(* Logix 5000 AddOnInstructionDefinition export Banner_iVu_VE_Functions; software revision 33.00 *)

TYPE Banner_iVu_VE_Control :   // Tags that control some basic functions of iVu and VE units.
STRUCT
   Reserved_PC : BOOL;   // Reserved for AOI internal use, to write to the VE input bit, for changing the running Inspection
   Reserved_TL : BOOL;   // Reserved for AOI internal use, to write to the VE input bit, For Match Teach, or Barcode Data Compare Teach
   Reserved_TR : BOOL;   // Reserved for AOI internal use, to write to the VE input bit, For triggering an image acquisition
   iVu_Command : BOOL;   // For iVu Command Channel over EIP only
   VE_Barcode_Data_Compare_Input_String : BOOL;   // For VE Barcode Data Compare only, saves a new compare string
   VE_FTP_Input_String : BOOL;   // For VE FTP file naming only, sends a new filename string
END_STRUCT
END_TYPE

TYPE Banner_iVu_VE_Data :   // Banner iVu and VE function data
STRUCT
   DTI : INT[17];   // Data Input Transfer Array
   DTO : INT[34];   // Data Output Transfer Array
   In : Banner_iVu_VE_Inputs;   // Input Data
   Out : Banner_iVu_VE_Outputs;   // Output Data
   Product_Change : BOOL;   // Tag that controls when a product change should be activated.
   Request_Product_Num : DINT;   // Tag in which the requested product change number is entered.
   Product_Change_Error : BOOL;   // Tag that states when a product change error has occurred.
   Teach : BOOL;   // Tag that controls when a teach should be activated.
   Teach_Request_Error : BOOL;   // Tag that states when a teach request error has occurred.
   Trigger : BOOL;   // Tag that controls when a trigger should be activated.
   Continuous_Trigger : BOOL;   // Tag that controls if triggering will be continuous or not.
   Trigger_Error : BOOL;   // Tag that states when a trigger error has occurred.
END_STRUCT
END_TYPE

TYPE Banner_iVu_VE_Input_Bits_Ack :
STRUCT
   Product_Change_Ack : BOOL;
   Teach_Latch_Ack : BOOL;
   Trigger_Ack : BOOL;
   iVu_Command_Ack : BOOL;
   VE_Barcode_Data_Compare_Input_String_Ack : BOOL;
   VE_FTP_Input_String_Ack : BOOL;
END_STRUCT
END_TYPE

TYPE Banner_iVu_VE_Inputs :
STRUCT
   Input_Bits_Ack : Banner_iVu_VE_Input_Bits_Ack;
   Output_Bits_Status : Banner_iVu_VE_Output_Status;
   Error_Code : DINT;
   Inspection_Num : DINT;
   Iteration_Count : DINT;
   Pass_Count : DINT;
   Fail_Count : DINT;
   Missed_Triggers : DINT;
   Current_Inspection_Time : REAL;
   Sensor_Pass_Fail : INT;
END_STRUCT
END_TYPE

TYPE Banner_iVu_VE_Output_Status :
STRUCT
   Ready : BOOL;
   Pass_Fail : BOOL;
   Read_No_Read_iVu : BOOL;   // (iVu BCR Only)
   Ready_to_Latch : BOOL;
   Output_1 : BOOL;
   Output_2 : BOOL;
   Output_3 : BOOL;
   Output_4_VE : BOOL;   // (VE Only)
   Output_5_VE : BOOL;   // (VE Only)
   Missed_Trigger : BOOL;
   Teach_Error : BOOL;
   System_Error : BOOL;
   Execution_Error : BOOL;
END_STRUCT
END_TYPE

TYPE Banner_iVu_VE_Outputs :
STRUCT
   Control_Registers : Banner_iVu_VE_Control;
   Reserved_PCN : DINT;   // Reserved for AOI Internal Use, to write the VE input value, for the requested product change inspection number
   VE_Input_String_Tool_Index : SINT;   // Specifies which Barcode tool in the VE Inspection should receive the string data (Optional)
   VE_Input_String : STRING_26;   // String for using as the barcode tool data compare Test string, or an FTP image file name
END_STRUCT
END_TYPE

TYPE STRING_26 :   // string type
STRUCT
   LEN : DINT;
   DATA : SINT[26];
END_STRUCT
END_TYPE

ADD_ON_INSTRUCTION Banner_iVu_VE_Convert_Data   (* revision 1.0 *)
VAR_IN_OUT
   Data : Banner_iVu_VE_Data; {required}
END_VAR

ROUTINE Logic   (* ladder *)
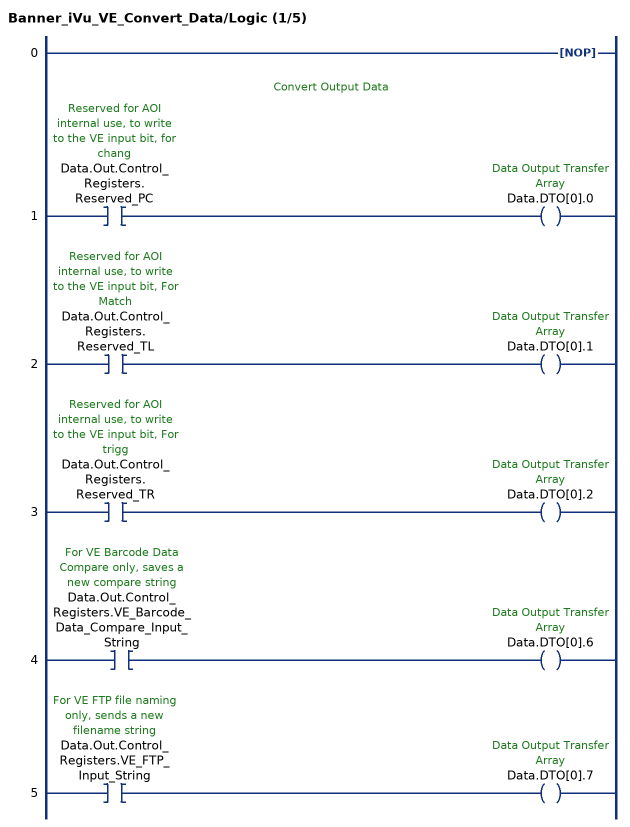
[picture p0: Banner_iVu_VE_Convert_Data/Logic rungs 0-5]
   0: NOP();
   // Convert Output Data
   1: XIC(Data.Out.Control_Registers.Reserved_PC)OTE(Data.DTO[0].0);
   2: XIC(Data.Out.Control_Registers.Reserved_TL)OTE(Data.DTO[0].1);
   3: XIC(Data.Out.Control_Registers.Reserved_TR)OTE(Data.DTO[0].2);
   4: XIC(Data.Out.Control_Registers.VE_Barcode_Data_Compare_Input_String)OTE(Data.DTO[0].6);
   5: XIC(Data.Out.Control_Registers.VE_FTP_Input_String)OTE(Data.DTO[0].7);
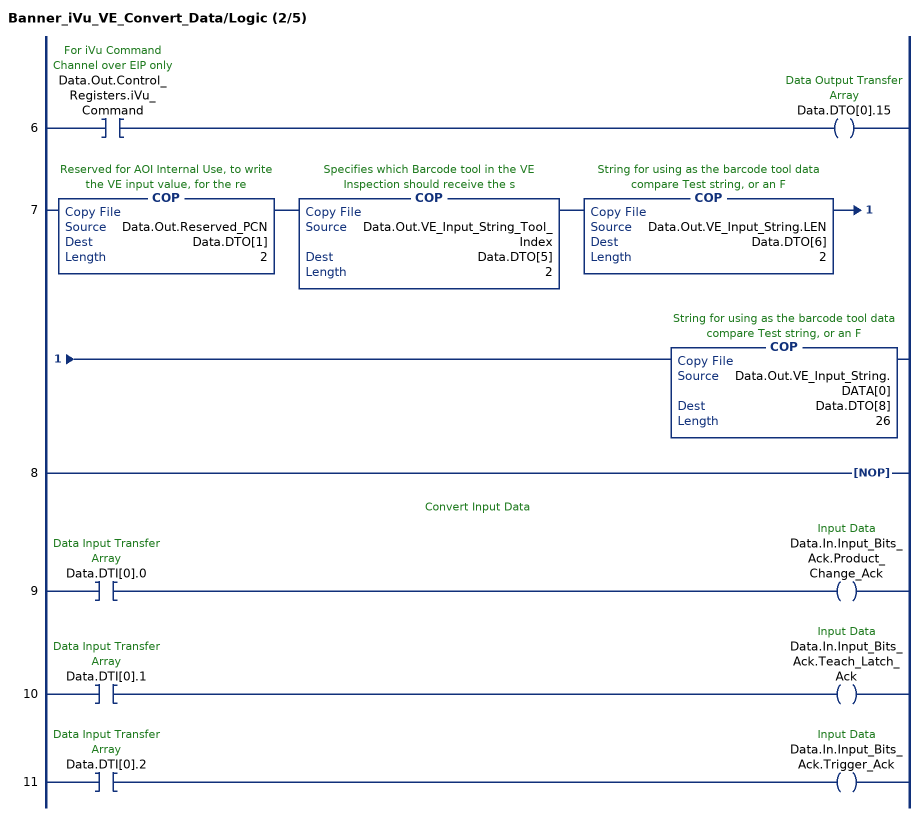
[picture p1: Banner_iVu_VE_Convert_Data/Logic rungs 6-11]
   6: XIC(Data.Out.Control_Registers.iVu_Command)OTE(Data.DTO[0].15);
   7: COP(Data.Out.Reserved_PCN,Data.DTO[1],2)COP(Data.Out.VE_Input_String_Tool_Index,Data.DTO[5],2)COP(Data.Out.VE_Input_String.LEN,Data.DTO[6],2)COP(Data.Out.VE_Input_String.DATA[0],Data.DTO[8],26);
   8: NOP();
   // Convert Input Data
   9: XIC(Data.DTI[0].0)OTE(Data.In.Input_Bits_Ack.Product_Change_Ack);
   10: XIC(Data.DTI[0].1)OTE(Data.In.Input_Bits_Ack.Teach_Latch_Ack);
   11: XIC(Data.DTI[0].2)OTE(Data.In.Input_Bits_Ack.Trigger_Ack);
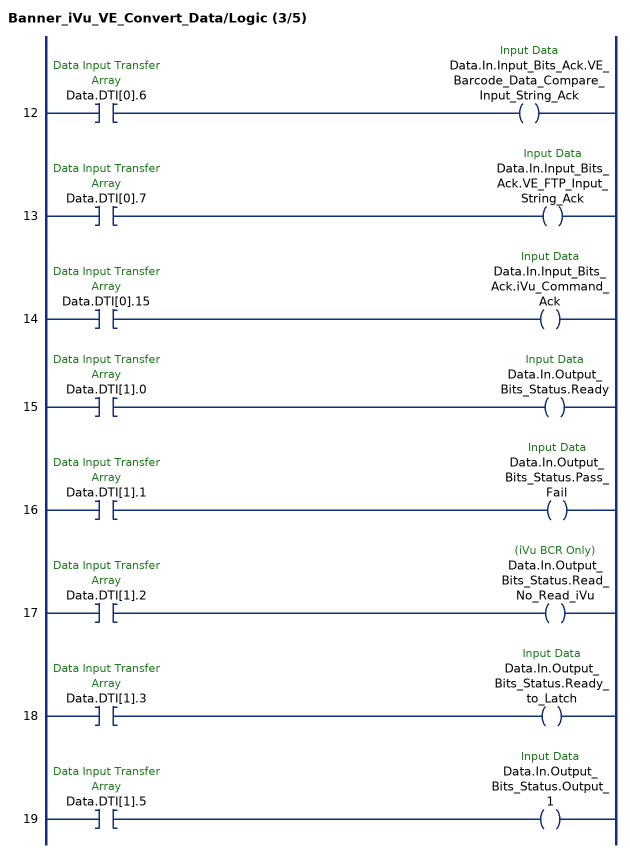
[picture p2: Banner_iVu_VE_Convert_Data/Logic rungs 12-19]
   12: XIC(Data.DTI[0].6)OTE(Data.In.Input_Bits_Ack.VE_Barcode_Data_Compare_Input_String_Ack);
   13: XIC(Data.DTI[0].7)OTE(Data.In.Input_Bits_Ack.VE_FTP_Input_String_Ack);
   14: XIC(Data.DTI[0].15)OTE(Data.In.Input_Bits_Ack.iVu_Command_Ack);
   15: XIC(Data.DTI[1].0)OTE(Data.In.Output_Bits_Status.Ready);
   16: XIC(Data.DTI[1].1)OTE(Data.In.Output_Bits_Status.Pass_Fail);
   17: XIC(Data.DTI[1].2)OTE(Data.In.Output_Bits_Status.Read_No_Read_iVu);
   18: XIC(Data.DTI[1].3)OTE(Data.In.Output_Bits_Status.Ready_to_Latch);
   19: XIC(Data.DTI[1].5)OTE(Data.In.Output_Bits_Status.Output_1);
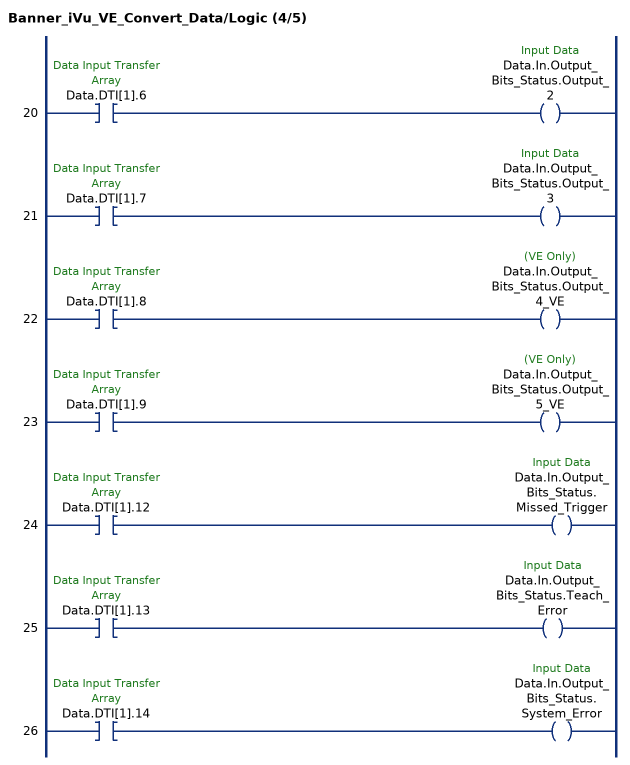
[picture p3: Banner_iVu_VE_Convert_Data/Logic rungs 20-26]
   20: XIC(Data.DTI[1].6)OTE(Data.In.Output_Bits_Status.Output_2);
   21: XIC(Data.DTI[1].7)OTE(Data.In.Output_Bits_Status.Output_3);
   22: XIC(Data.DTI[1].8)OTE(Data.In.Output_Bits_Status.Output_4_VE);
   23: XIC(Data.DTI[1].9)OTE(Data.In.Output_Bits_Status.Output_5_VE);
   24: XIC(Data.DTI[1].12)OTE(Data.In.Output_Bits_Status.Missed_Trigger);
   25: XIC(Data.DTI[1].13)OTE(Data.In.Output_Bits_Status.Teach_Error);
   26: XIC(Data.DTI[1].14)OTE(Data.In.Output_Bits_Status.System_Error);
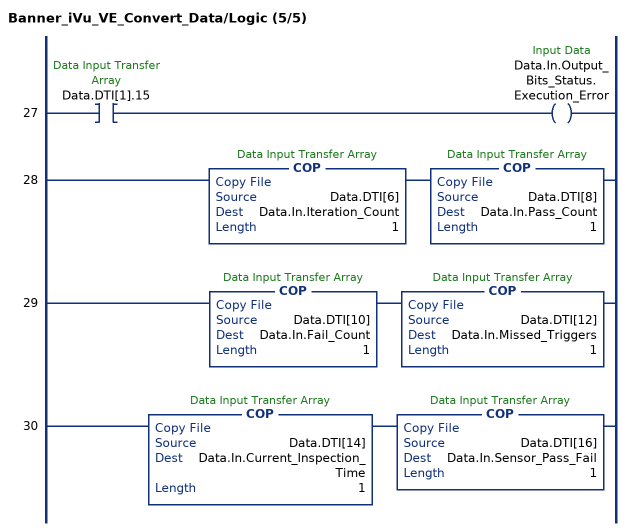
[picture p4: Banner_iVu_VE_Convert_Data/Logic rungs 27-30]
   27: XIC(Data.DTI[1].15)OTE(Data.In.Output_Bits_Status.Execution_Error);
   28: COP(Data.DTI[6],Data.In.Iteration_Count,1)COP(Data.DTI[8],Data.In.Pass_Count,1);
   29: COP(Data.DTI[10],Data.In.Fail_Count,1)COP(Data.DTI[12],Data.In.Missed_Triggers,1);
   30: COP(Data.DTI[14],Data.In.Current_Inspection_Time,1)COP(Data.DTI[16],Data.In.Sensor_Pass_Fail,1);
END_ROUTINE
END_ADD_ON_INSTRUCTION

ADD_ON_INSTRUCTION Banner_Vision_Product_Change   (* revision 1.0, vendor Banner Engineering *)
// Instruction to do a product change for a iVu or VE vision sensor.
VAR_INPUT
   Ready_Bit : BOOL; {required}   // Bit that determines status of the Vision Sensor.
   Product_Change_ACK_Bit : BOOL; {required}   // Bit that states the Acknowledgement Bit Status.
   Requested_Product_Number : INT; {required}   // Product Number that the PLC is requesting.
   System_Error_Bit : BOOL; {required}   // Status of the System Error Bit.
   Execution_Error_Bit : BOOL; {required}   // Status of the Execution Error Bit.
END_VAR
VAR_IN_OUT
   Error_Output : BOOL; {required}   // If the Product Change fails activate an Error Bit so the PLC can solve the error.
   Product_Change_Bit : BOOL; {required}   // Bit that controls the Product Change proces.
   Product_Change_Control_Bit : BOOL; {required}   // Bit that controls the Product Change routine.
   Product_Change_Number : DINT; {required}   // Inspection number that the Vision sensor should change to.
END_VAR
VAR
   Lock_2 : BOOL; {access None}
   Ladder_Control_Bit : BOOL; {access None}
   Timer : TIMER := (PRE := 50); {access None}
END_VAR

ROUTINE Logic   (* ladder *)
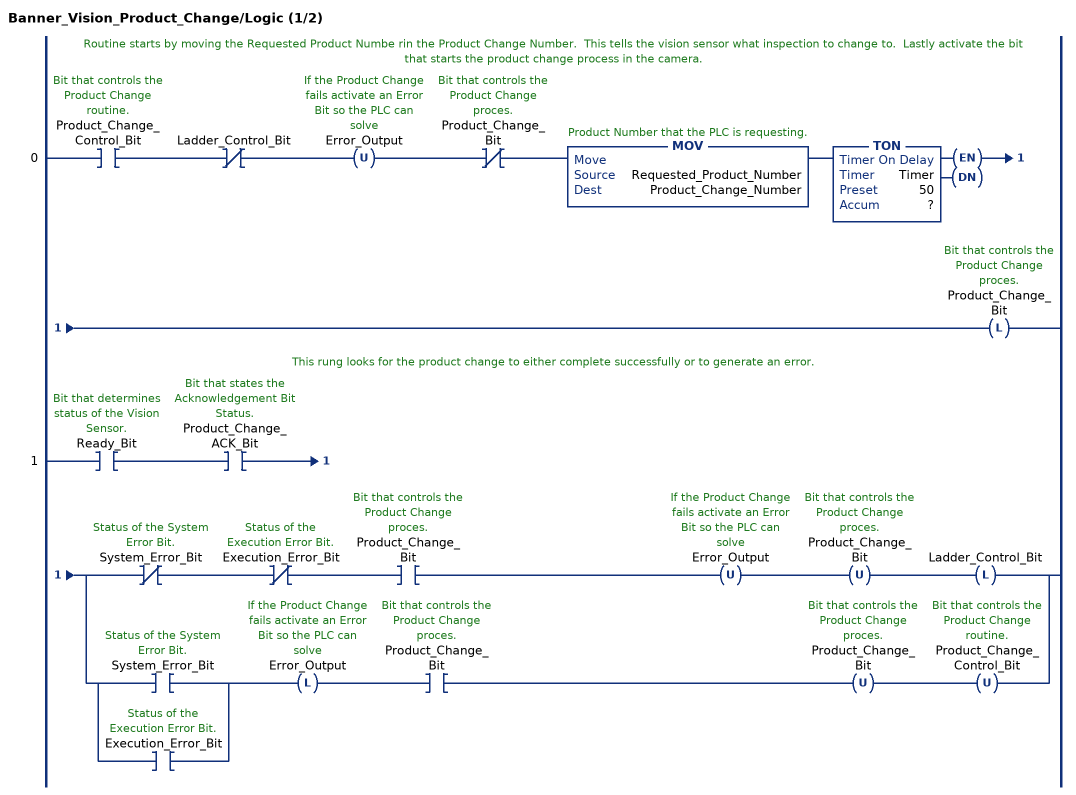
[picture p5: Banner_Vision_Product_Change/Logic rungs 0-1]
   // Routine starts by moving the Requested Product Numbe rin the Product Change Number.  This tells the vision sensor what inspection to change to.  Lastly activate the bit that starts the product change process in the camera.
   0: XIC(Product_Change_Control_Bit)XIO(Ladder_Control_Bit)OTU(Error_Output)XIO(Product_Change_Bit)MOV(Requested_Product_Number,Product_Change_Number)TON(Timer,?,?)OTL(Product_Change_Bit);
   // This rung looks for the product change to either complete successfully or to generate an error.
   1: XIC(Ready_Bit)XIC(Product_Change_ACK_Bit)[XIO(System_Error_Bit) XIO(Execution_Error_Bit) XIC(Product_Change_Bit) OTU(Error_Output) OTU(Product_Change_Bit) OTL(Ladder_Control_Bit) ,[XIC(System_Error_Bit) ,XIC(Execution_Error_Bit) ] OTL(Error_Output) XIC(Product_Change_Bit) OTU(Product_Change_Bit) OTU(Product_Change_Control_Bit) ];
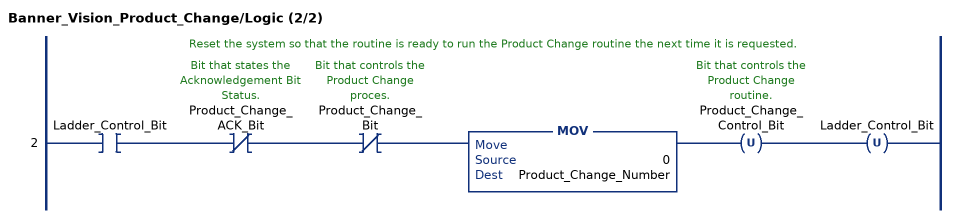
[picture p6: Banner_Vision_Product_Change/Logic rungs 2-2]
   // Reset the system so that the routine is ready to run the Product Change routine the next time it is requested.
   2: XIC(Ladder_Control_Bit)XIO(Product_Change_ACK_Bit)XIO(Product_Change_Bit)MOV(0,Product_Change_Number)OTU(Product_Change_Control_Bit)OTU(Ladder_Control_Bit);
END_ROUTINE
END_ADD_ON_INSTRUCTION

ADD_ON_INSTRUCTION Banner_Vision_Teach   (* revision 1.0, vendor Banner Engineering *)
// Instruction to request a Teach for a iVu or VE vision sensor.
VAR_INPUT
   Teach_Ack_Bit : BOOL; {required}   // Status of the Teach Acknowledgement bit.
   Ready_Bit : BOOL; {required}   // Status of the Camera Ready bit.
   Execution_Error : BOOL; {required}   // Status of the Execution Error from the Vision Sensor.
   System_Error : BOOL; {required}   // Status of the System Error from the Vision Sensor.
   Teach_Error : BOOL; {required}   // Status of the Teach Error from the Vision Sensor.
END_VAR
VAR_IN_OUT
   Teach_Error_Output : BOOL; {required}   // When an error in the Teach routine is detected activated this bit so the PLC can begin a recovery routine.
   Teach_Control_Bit : BOOL; {required}   // Bit that controls the activation of the Teach AOI.
   Teach_Bit : BOOL; {required}   // Bit that controls the activation of the Teach routine in the vision sensor.
END_VAR
VAR
   Ladder_Control_2 : BOOL; {access None}
   Ladder_Control_1 : BOOL; {access None}
END_VAR

ROUTINE Logic   (* ladder *)
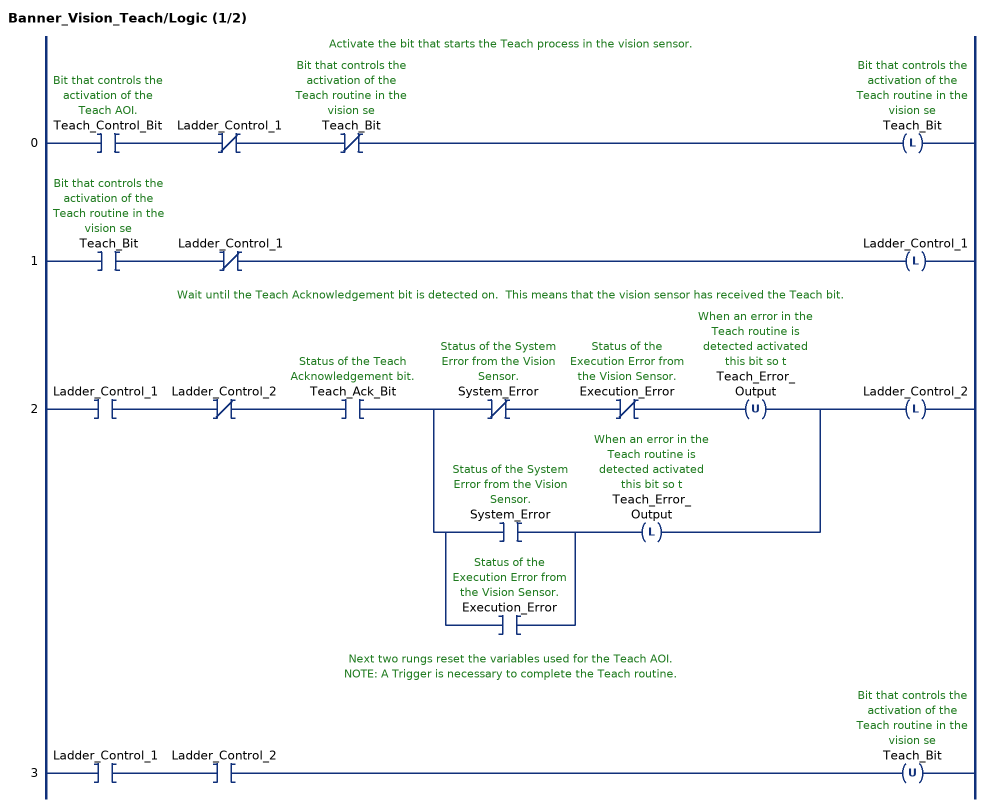
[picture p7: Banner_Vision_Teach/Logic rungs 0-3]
   // Activate the bit that starts the Teach process in the vision sensor.
   0: XIC(Teach_Control_Bit)XIO(Ladder_Control_1)XIO(Teach_Bit)OTL(Teach_Bit);
   1: XIC(Teach_Bit)XIO(Ladder_Control_1)OTL(Ladder_Control_1);
   // Wait until the Teach Acknowledgement bit is detected on.  This means that the vision sensor has received the Teach bit.
   2: XIC(Ladder_Control_1)XIO(Ladder_Control_2)XIC(Teach_Ack_Bit)[XIO(System_Error) XIO(Execution_Error) OTU(Teach_Error_Output) ,[XIC(System_Error) ,XIC(Execution_Error) ] OTL(Teach_Error_Output) ]OTL(Ladder_Control_2);
   // Next two rungs reset the variables used for the Teach AOI.
   // NOTE: A Trigger is necessary to complete the Teach routine.
   3: XIC(Ladder_Control_1)XIC(Ladder_Control_2)OTU(Teach_Bit);
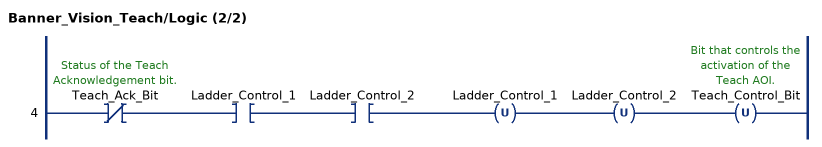
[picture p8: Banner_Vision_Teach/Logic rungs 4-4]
   4: XIO(Teach_Ack_Bit)XIC(Ladder_Control_1)XIC(Ladder_Control_2)OTU(Ladder_Control_1)OTU(Ladder_Control_2)OTU(Teach_Control_Bit);
END_ROUTINE
END_ADD_ON_INSTRUCTION

ADD_ON_INSTRUCTION Banner_Vision_Trigger   (* revision 1.0, vendor Banner Engineering *)
// Instruction to do a Trigger for a iVu or VE vision sensor.
VAR_INPUT
   Ready_Bit : BOOL; {required}   // Status of the Ready Bit from the Vision Sensor.
   Trigger_Ack_Bit : BOOL; {required}   // Status of the Trigger Acknowledgement Bit.
   System_Error : BOOL; {required}   // Status of the System Error from the Vision Sensor.
   Execution_Error : BOOL; {required}   // Status of the Execution Error from the Vision Sensor.
END_VAR
VAR_IN_OUT
   Trigger_Error : BOOL; {required}   // The Trigger Error bit is activated when the AOI detects an error from the Vision Sensor.
   Trigger_Bit : BOOL; {required}   // Trigger Bit controls the activation of a Trigger in the Vision Sensor.
   Trigger_Control : BOOL; {required}   // Bit that controls the activation of the Vision Trigger AOI.
END_VAR
VAR
   Ladder_Control : BOOL; {access None}
END_VAR

ROUTINE Logic   (* ladder *)
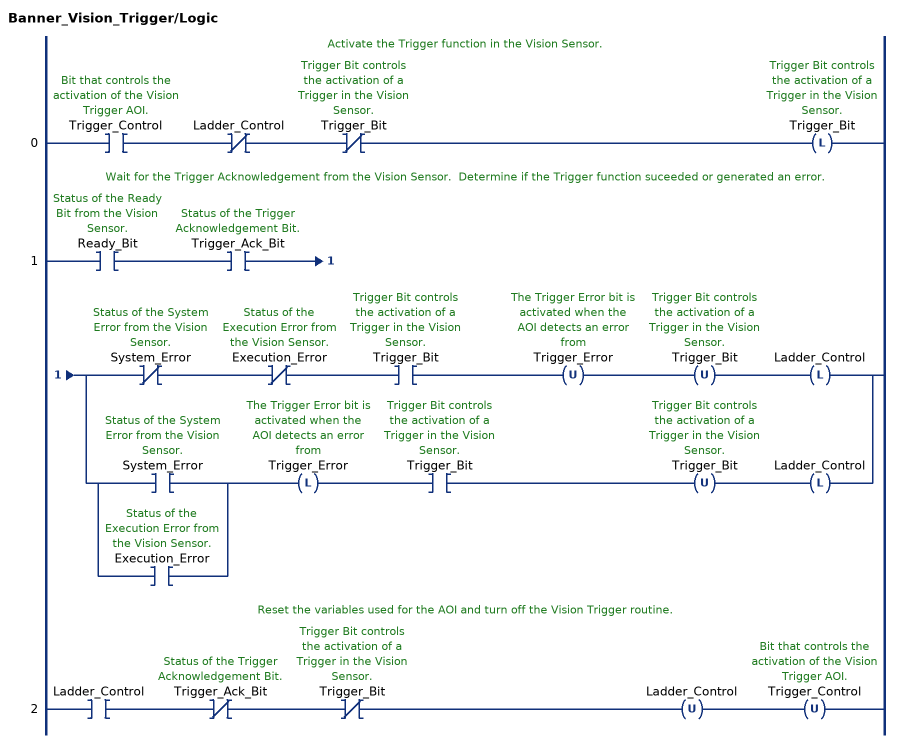
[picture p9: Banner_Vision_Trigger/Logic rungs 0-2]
   // Activate the Trigger function in the Vision Sensor.
   0: XIC(Trigger_Control)XIO(Ladder_Control)XIO(Trigger_Bit)OTL(Trigger_Bit);
   // Wait for the Trigger Acknowledgement from the Vision Sensor.  Determine if the Trigger function suceeded or generated an error.
   1: XIC(Ready_Bit)XIC(Trigger_Ack_Bit)[XIO(System_Error) XIO(Execution_Error) XIC(Trigger_Bit) OTU(Trigger_Error) OTU(Trigger_Bit) OTL(Ladder_Control) ,[XIC(System_Error) ,XIC(Execution_Error) ] OTL(Trigger_Error) XIC(Trigger_Bit) OTU(Trigger_Bit) OTL(Ladder_Control) ];
   // Reset the variables used for the AOI and turn off the Vision Trigger routine.
   2: XIC(Ladder_Control)XIO(Trigger_Ack_Bit)XIO(Trigger_Bit)OTU(Ladder_Control)OTU(Trigger_Control);
END_ROUTINE
END_ADD_ON_INSTRUCTION

ADD_ON_INSTRUCTION Banner_iVu_VE_Functions   (* revision 2.4 *)
// AOI to allow for the basic functions of a Banner iVu or VE device.
// Revision note:
// Replaced BTD commands with COP commands to reduce the instruction count, and moved a contact in the Product Change subroutine.
VAR_IN_OUT
   Data : Banner_iVu_VE_Data; {required}
END_VAR
VAR
   Lock : DINT; {access None}
   Vision_Teach : Banner_Vision_Teach; {access None}
   Vision_Trigger : Banner_Vision_Trigger; {access None}
   Vision_Product : Banner_Vision_Product_Change; {access None}
   Temp_Change : DINT; {access None}
   Convert_Status : Banner_iVu_VE_Convert_Data; {access None}
END_VAR

ROUTINE Logic   (* ladder *)
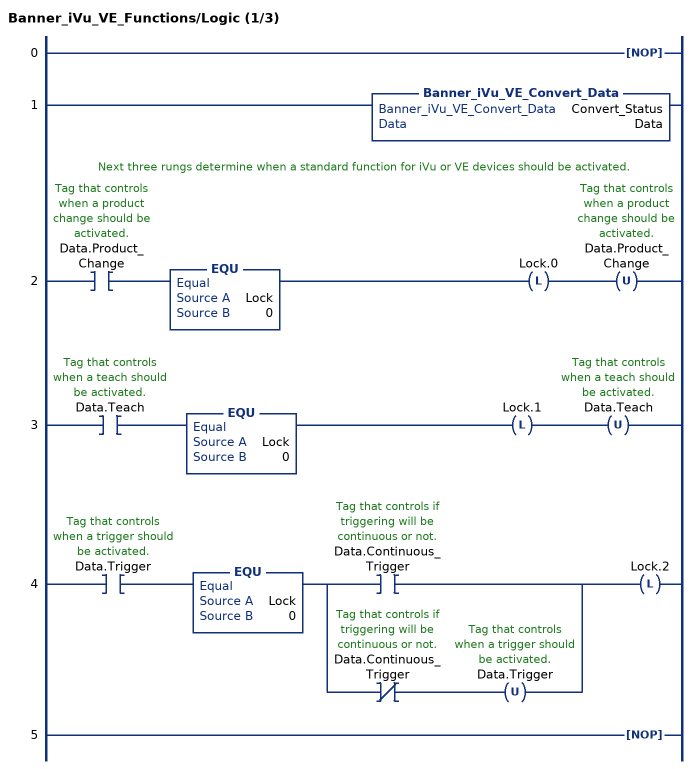
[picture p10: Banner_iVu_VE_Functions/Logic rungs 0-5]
   0: NOP();
   1: Banner_iVu_VE_Convert_Data(Convert_Status,Data);
   // Next three rungs determine when a standard function for iVu or VE devices should be activated.
   2: XIC(Data.Product_Change)EQU(Lock,0)OTL(Lock.0)OTU(Data.Product_Change);
   3: XIC(Data.Teach)EQU(Lock,0)OTL(Lock.1)OTU(Data.Teach);
   4: XIC(Data.Trigger)EQU(Lock,0)[XIC(Data.Continuous_Trigger) ,XIO(Data.Continuous_Trigger) OTU(Data.Trigger) ]OTL(Lock.2);
   5: NOP();
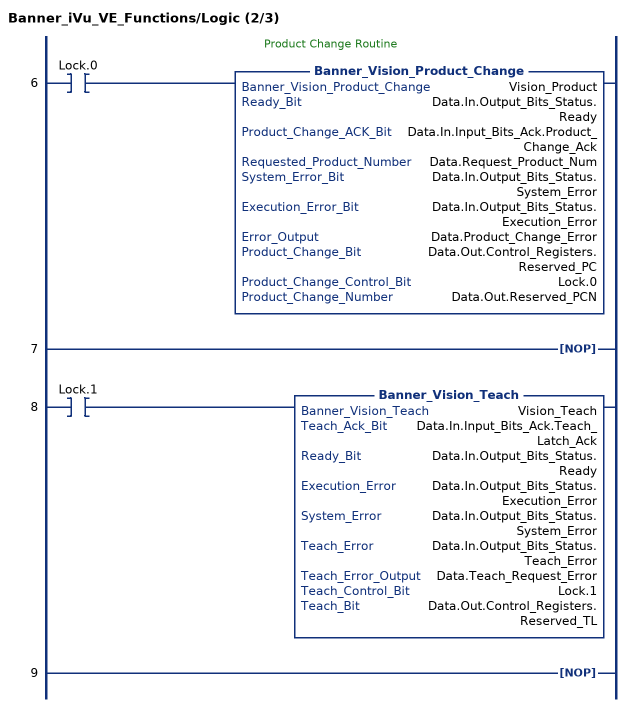
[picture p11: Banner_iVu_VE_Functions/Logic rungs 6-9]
   // Product Change Routine
   6: XIC(Lock.0)Banner_Vision_Product_Change(Vision_Product,Data.In.Output_Bits_Status.Ready,Data.In.Input_Bits_Ack.Product_Change_Ack,Data.Request_Product_Num,Data.In.Output_Bits_Status.System_Error,Data.In.Output_Bits_Status.Execution_Error,Data.Product_Change_Error,Data.Out.Control_Registers.Reserved_PC,Lock.0,Data.Out.Reserved_PCN);
   7: NOP();
   8: XIC(Lock.1)Banner_Vision_Teach(Vision_Teach,Data.In.Input_Bits_Ack.Teach_Latch_Ack,Data.In.Output_Bits_Status.Ready,Data.In.Output_Bits_Status.Execution_Error,Data.In.Output_Bits_Status.System_Error,Data.In.Output_Bits_Status.Teach_Error,Data.Teach_Request_Error,Lock.1,Data.Out.Control_Registers.Reserved_TL);
   9: NOP();
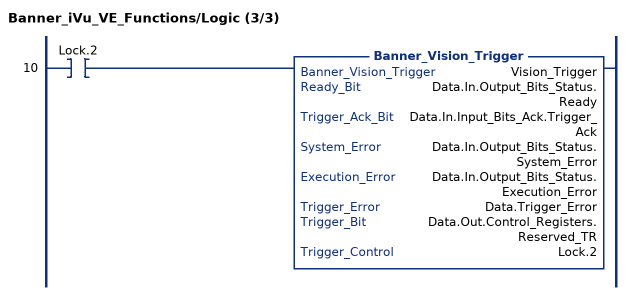
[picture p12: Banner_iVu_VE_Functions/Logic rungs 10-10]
   10: XIC(Lock.2)Banner_Vision_Trigger(Vision_Trigger,Data.In.Output_Bits_Status.Ready,Data.In.Input_Bits_Ack.Trigger_Ack,Data.In.Output_Bits_Status.System_Error,Data.In.Output_Bits_Status.Execution_Error,Data.Trigger_Error,Data.Out.Control_Registers.Reserved_TR,Lock.2);
END_ROUTINE
END_ADD_ON_INSTRUCTION
